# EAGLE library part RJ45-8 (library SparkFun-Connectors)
RJ45 Jack - 8 pin Simple RJ45, 8-pin connection. Commonly used for Cat5, Cat5e, and Cat6 Ethernet cables. Here is the connector we sell at SparkFun: RJ45 8-Pin Connector (PRT-00643) Datasheet It is used on this SparkFun product: SparkFun RJ45 Breakout (BOB-00716) Note, you may also be interested in the "MAGJACK" version of this. It is basically a RJ45 connector, but also has some status LEDs built into the connector housing. You can check that out in this library at the device named "MAGJACK.dev" and see these products online: RJ45 Ethernet MagJack-Compatible (PRT-08534) SparkFun RJ45 MagJack Breakout (BOB-13021)
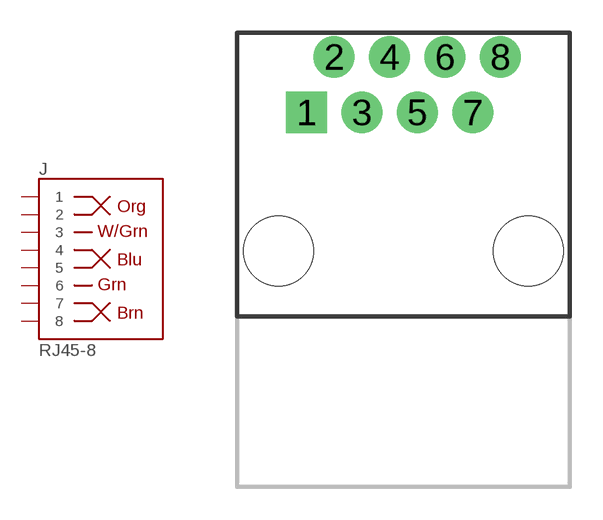
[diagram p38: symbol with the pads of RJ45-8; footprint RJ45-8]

Designator prefix J

## RJ45-8 (PROD_ID: CONN-08506; SF_ID: PRT-00643; VALUE: RJ45)  [RJ45-8]
1  1
2  2
3  3
4  4
5  5
6  6
7  7
8  8

## Footprint RJ45-8 (pad centres in mm)
RJ45 Socket with PCB Mounting Posts Specifications: Pin count:8 Datasheet referenced for footprint Example device(s): RJ45-8
drill 1 pad 1.88 square: 1 -4.445,6.35
drill 1 pad 1.88: 2 -3.175,8.89; 3 -1.905,6.35; 4 -0.635,8.89; 5 0.635,6.35; 6 1.905,8.89; 7 3.175,6.35; 8 4.445,8.89
hole 3.2 at -5.715,0
hole 3.2 at 5.715,0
